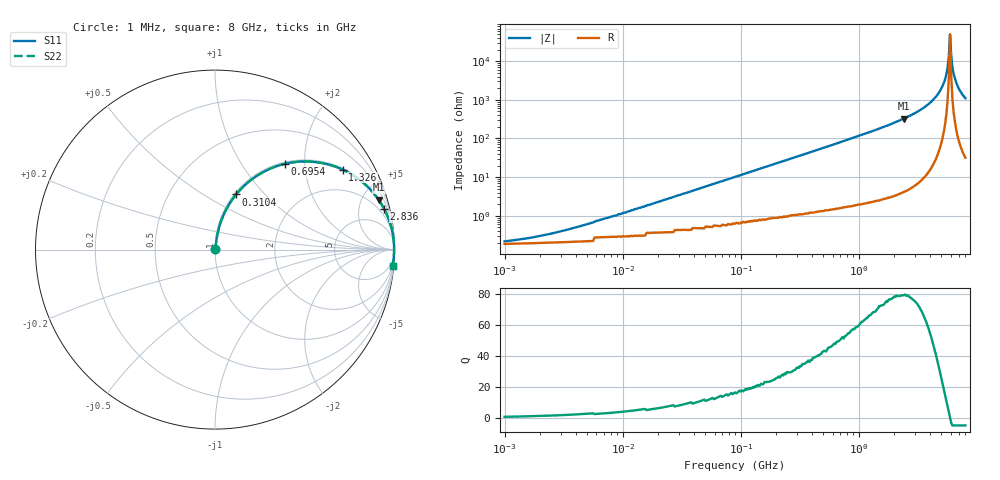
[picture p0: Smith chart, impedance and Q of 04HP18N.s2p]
# MHz S MA R 50
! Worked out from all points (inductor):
!   391 points, 1 MHz to 8 GHz, reference 50 ohm
!   read as one part in series: L = 18 nH near 7.598 MHz
!   highest Q = 79.1 at 2.414 GHz (marker M1), where L = 21.6 nH
!   self-resonance near 5.929 GHz
!   S11 on the Smith chart (normalised r, x): 1 MHz: 1.00, +0.00; 310.4 MHz: 1.02, +0.70; 695.4 MHz: 1.03, +1.60; 1.326 GHz: 1.05, +3.16; 2.836 GHz: 1.12, +8.31; 8 GHz: 2, -22
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1  0.002072 33.0  0.998 -0.1  0.998 -0.1  0.002072 33.0
4.576  0.005673 65.2  0.998 -0.3  0.998 -0.3  0.005673 65.2
20.466  0.023 79.7  0.996 -1.3  0.996 -1.3  0.023 79.7
89.443  0.1 80.7  0.989 -5.7  0.989 -5.7  0.1 80.7
310.437  0.329 69.0  0.934 -19.2  0.934 -19.2  0.329 69.0
409.325  0.418 63.8  0.898 -24.7  0.898 -24.7  0.418 63.8
695.425  0.618 50.7  0.774 -38.1  0.774 -38.1  0.618 50.7
1325.782  0.839 32.1  0.532 -57.0  0.532 -57.0  0.839 32.1
1830.556  0.912 23.5  0.399 -65.8  0.399 -65.8  0.912 23.5
2413.671  0.953 16.9  0.291 -72.3  0.291 -72.3  0.953 16.9
2836.178  0.969 13.5  0.233 -75.8  0.233 -75.8  0.969 13.5
4100.721  0.992 6.4  0.112 -82.5  0.112 -82.5  0.992 6.4
5045.817  0.997 2.8  0.048 -84.9  0.048 -84.9  0.997 2.8
5406.987  0.998 1.6  0.028 -84.3  0.028 -84.3  0.998 1.6
5662.017  0.998 0.8  0.014 -81.0  0.014 -81.0  0.998 0.8
5794.008  0.998 0.4  0.007258 -73.5  0.007258 -73.5  0.998 0.4
5929.076  0.998 0.0  0.002034 -3.3  0.002034 -3.3  0.998 0.0
6067.292  0.998 -0.4  0.007044 72.7  0.007044 72.7  0.998 -0.4
6208.731  0.998 -0.8  0.014 80.5  0.014 80.5  0.998 -0.8
6353.467  0.998 -1.2  0.021 83.0  0.021 83.0  0.998 -1.2
6966.946  0.997 -2.8  0.048 84.6  0.048 84.6  0.997 -2.8
8000  0.993 -5.2  0.09 83.2  0.09 83.2  0.993 -5.2
